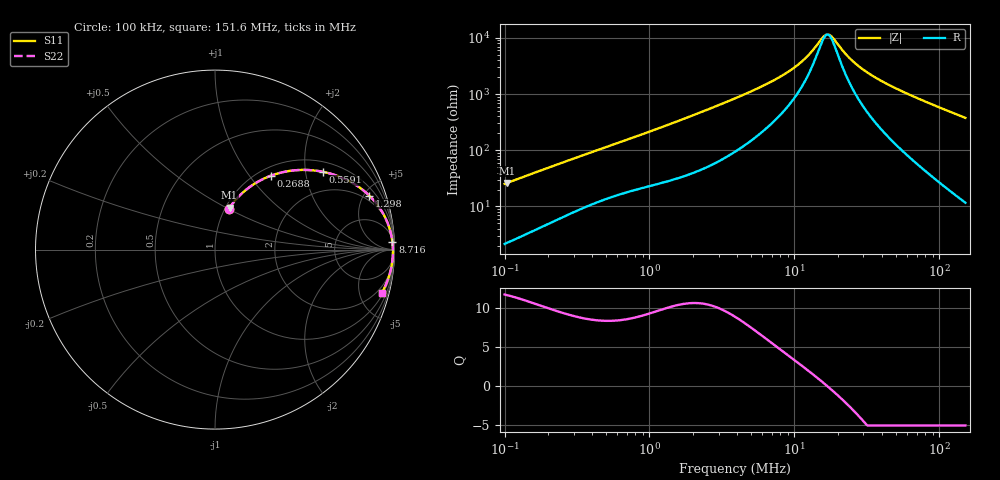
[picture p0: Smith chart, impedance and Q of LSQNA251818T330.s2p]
! LSQNA251818T330  S-PARAMETER MODEL  ( General Type )
! Model Generated by TAIYO YUDEN Corporation (http://www.ty-top.com)
! Version 2.0
! TAIYO YUDEN Control No. 100810NF25SB-FKC
! Copyright(c) 2007 TAIYO YUDEN CO.,LTD. All Rights Reserved.
! Product Description (link to TY-COMPAS)
! https://ds.yuden.co.jp/TYCOMPAS/or/detail?pn=LSQNA251818T330K&u=M
! Products Name : Inductors
! Characteristics :
!  Inductance : 33 uH , SRF(min) : 15 MHz , DC Resistance(max) : 0.91 Ohm
!  Rated Current : Saturation :130 mA , Temp Rise : 460 mA (40 degC)
!  Case Size : 2.5 x 1.8 / 0.098 x 0.071 [mm/inch] , Thickness : 1.8 / 0.071 [mm/inch]
!  (Conditions: Temperature = 25 degC , DC Bias Current/Voltage = 0A / 0V)
! External Node Assignments :
!  1  o---GGG---o  2
! GND o---------o GND
! Frequency Range : 0.1MHz  -  151.640846MHz  [ 402 STEP ]
# MHz S RI R 50
! Freq[MHz].  S11 Real  S11 Imag  S21 Real  S21 Imag  S12 Real  S12 Imag  S22 Real  S22 Imag
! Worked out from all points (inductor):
!   401 points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, 100 kHz to 151.6 MHz, reference 50 ohm
!   read as one part in series: L = 39.6 uH near 103.7 kHz
!   highest Q = 11.6 at 103.7 kHz (marker M1), where L = 40 uH
!   self-resonance near 16.85 MHz
!   S11 on the Smith chart (normalised r, x): 100 kHz: 1.04, +0.50; 268.8 kHz: 1.14, +1.28; 559.1 kHz: 1.30, +2.49; 1.298 MHz: 1.55, +5.46; 8.716 MHz: 12, +45; 151.6 MHz: 1.23, -7.53
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0.1  0.077 0.2272  0.923 -0.2272  0.923 -0.2272  0.077 0.2272
0.10373  0.0815 0.234  0.9185 -0.234  0.9185 -0.234  0.0815 0.234
0.166977  0.1675 0.3286  0.8325 -0.3286  0.8325 -0.3286  0.1675 0.3286
0.268788  0.3115 0.4119  0.6885 -0.4119  0.6885 -0.4119  0.3115 0.4119
0.341025  0.402 0.4362  0.598 -0.4362  0.598 -0.4362  0.402 0.4362
0.559103  0.6002 0.4336  0.3998 -0.4336  0.3998 -0.4336  0.6002 0.4336
1.162983  0.8353 0.3227  0.1647 -0.3227  0.1647 -0.3227  0.8353 0.3227
1.298033  0.8598 0.3006  0.1402 -0.3006  0.1402 -0.3006  0.8598 0.3006
2.128094  0.9348 0.2041  0.0652 -0.2041  0.0652 -0.2041  0.9348 0.2041
3.894109  0.9735 0.1139  0.0265 -0.1139  0.0265 -0.1139  0.9735 0.1139
6.154731  0.9845 0.0674  0.0155 -0.0674  0.0155 -0.0674  0.9845 0.0674
8.715612  0.9884 0.0408  0.0116 -0.0408  0.0116 -0.0408  0.9884 0.0408
11.05795  0.99 0.0253  0.00999 -0.0253  0.00999 -0.0253  0.99 0.0253
13.2799  0.9908 0.0142  0.00919 -0.0142  0.00919 -0.0142  0.9908 0.0142
15.94833  0.9913 0.00346  0.0087 -0.00346  0.0087 -0.00346  0.9913 0.00346
17.47734  0.9914 -0.00187  0.00856 0.00187  0.00856 0.00187  0.9914 -0.00187
23.00149  0.9914 -0.0182  0.00857 0.0182  0.00857 0.0182  0.9914 -0.0182
26.63007  0.9911 -0.0275  0.00886 0.0275  0.00886 0.0275  0.9911 -0.0275
33.78694  0.9901 -0.0439  0.00989 0.0439  0.00989 0.0439  0.9901 -0.0439
45.28783  0.9875 -0.0675  0.0125 0.0675  0.0125 0.0675  0.9875 -0.0675
78.44093  0.9754 -0.1281  0.0246 0.1281  0.0246 0.1281  0.9754 -0.1281
151.6408  0.9277 -0.2441  0.0723 0.2441  0.0723 0.2441  0.9277 -0.2441
